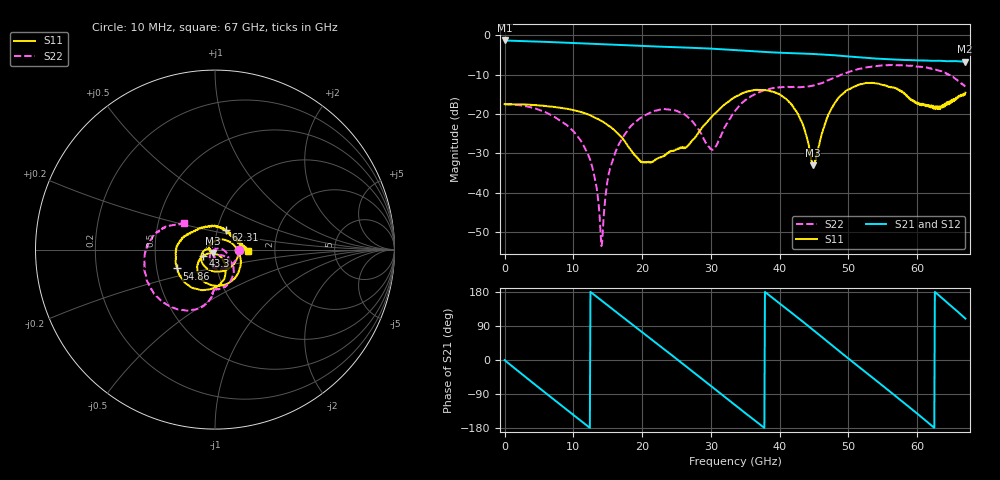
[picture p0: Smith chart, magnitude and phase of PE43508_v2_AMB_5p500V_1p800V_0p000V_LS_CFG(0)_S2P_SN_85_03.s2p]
!Keysight Technologies,N5227A,US51270237,A.10.43.00
!Date: Wednesday, August 22, 2018 17:06:30
!Correction: S11(Full 2 Port(1,3))
!S31(Full 2 Port(1,3))
!S13(Full 2 Port(1,3))
!S33(Full 2 Port(1,3))
!S2P File: Measurements: S11, S31, S13, S33:
# Hz S  dB  R 50
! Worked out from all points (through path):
!   801 points, 10 MHz to 67 GHz, reference 50 ohm
!   highest |S21| = -1.33 dB at 10 MHz (marker M1); lowest = -6.7 dB at 66.92 GHz (marker M2)
!   group delay of S21, straight-line fit = 39.9 ps
!   lowest |S11| = -33.0 dB at 44.81 GHz (marker M3), VSWR 1.05, Z = 48.9 - j1.9 ohm
!   |S11| at or under -10 dB: start of sweep to end of sweep
!   |S22| runs from -53.5 to -7.5 dB; largest |S21 - S12| = 0.0053
!   S11 on the Smith chart (normalised r, x): 10 MHz: 1.31, -0.00; 43.3 GHz: 0.87, -0.06; 54.86 GHz: 0.64, -0.14; 62.31 GHz: 1.10, +0.25; 67 GHz: 1.46, -0.03
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1e7  -17.47 -0.5  -1.33 -0.2  -1.33 -0.2  -17.48 -0.7
5.70415e9  -17.91 -70.8  -1.67 -83.3  -1.67 -83.3  -19.36 -69.6
1.123082e10  -19.55 -129.7  -2.05 -162.4  -2.05 -162.3  -27.10 -130.3
1.290558e10  -20.68 -146.5  -2.18 173.8  -2.17 173.8  -34.54 -150.5
1.416164e10  -21.83 -158.3  -2.27 156.0  -2.26 156.1  -53.00 91.0
1.516649e10  -23.00 -167.9  -2.34 141.8  -2.34 141.8  -35.04 19.0
1.650629e10  -25.03 -178.5  -2.45 122.8  -2.44 122.8  -28.05 3.5
1.935336e10  -31.15 177.3  -2.66 82.6  -2.65 82.6  -21.54 -28.5
2.236791e10  -31.14 -161.3  -2.88 40.1  -2.87 40.1  -18.96 -60.3
2.61361e10  -28.45 132.1  -3.12 -13.1  -3.11 -13.2  -20.04 -96.4
3.023924e10  -20.41 26.0  -3.43 -71.9  -3.42 -71.8  -28.98 -67.2
3.3505e10  -15.70 -29.4  -3.75 -118.7  -3.74 -118.6  -19.21 -37.1
3.81943e10  -14.00 -94.5  -4.28 174.9  -4.27 174.9  -13.81 -68.4
4.330229e10  -22.41 -151.7  -4.64 102.1  -4.64 102.1  -13.13 -90.9
4.472582e10  -32.24 -127.4  -4.74 81.3  -4.73 81.4  -12.82 -92.0
4.480956e10  -33.00 -119.9  -4.75 80.1  -4.73 80.1  -12.80 -91.9
4.857775e10  -15.83 -70.1  -5.17 24.6  -5.18 24.5  -10.33 -99.3
5.485806e10  -12.54 -153.7  -6.00 -66.2  -5.98 -66.5  -7.69 -136.0
5.586291e10  -13.14 -169.2  -6.09 -80.9  -6.09 -81.2  -7.57 -142.3
6.23107e10  -17.89 61.3  -6.50 -176.5  -6.53 -176.6  -8.59 174.8
6.691626e10  -15.10 -1.4  -6.71 110.6  -6.76 110.9  -12.90 141.2
6.7e10  -14.58 -3.2  -6.70 109.3  -6.74 109.5  -12.98 139.5
